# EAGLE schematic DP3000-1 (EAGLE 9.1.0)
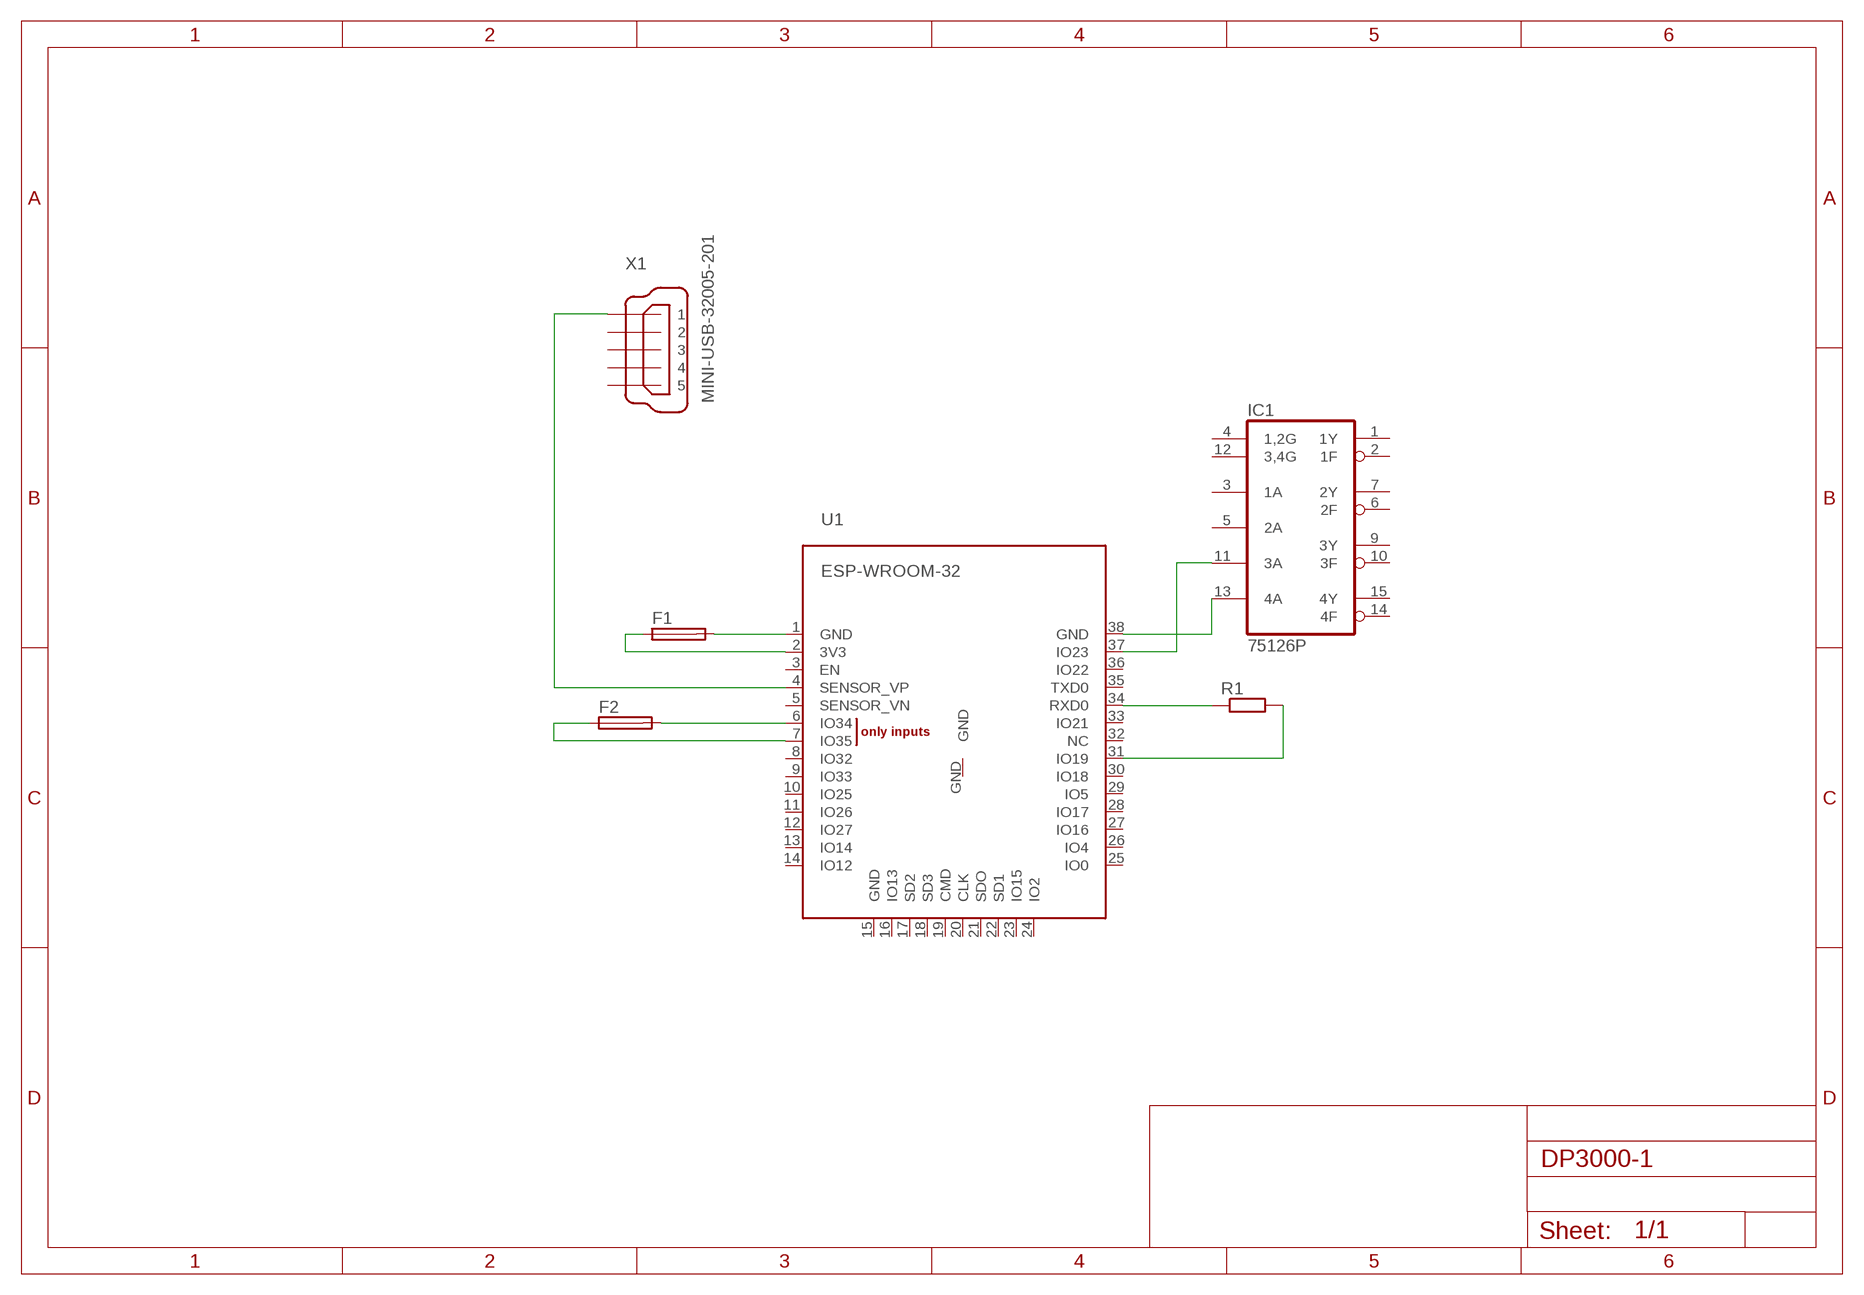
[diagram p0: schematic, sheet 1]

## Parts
F1  19560  [19560]
F2  KS16  [KS16]
IC1  75126P  [DIL16]
R1  R-EU_R2012  [R2012]
U1  ESP-WROOM-32  [ESP-WROOM-32]
X1  MINI-USB-32005-201  [32005-201]

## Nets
N$1: R1.1 U1.34(RXD0)
N$2: R1.2 U1.31(IO19)
N$3: IC1.13(4A) U1.38(GND)
N$4: IC1.11(3A) U1.37(IO23)
N$5: F1.2 U1.1(GND)
N$6: F1.1 U1.2(3V3)
N$7: F2.2 U1.6(IO34)
N$8: F2.1 U1.7(IO35)
N$9: U1.4(SENSOR_VP) X1.1
Unconnected: IC1.1(1Y) IC1.2(1F) IC1.3(1A) IC1.4(1,2G) IC1.5(2A) IC1.6(2F) IC1.7(2Y) IC1.9(3Y) IC1.10(3F) IC1.12(3,4G) IC1.14(4F) IC1.15(4Y) U1.3(EN) U1.5(SENSOR_VN) U1.8(IO32) U1.9(IO33) U1.10(IO25) U1.11(IO26) U1.12(IO27) U1.13(IO14) U1.14(IO12) U1.15(GND) U1.16(IO13) U1.17(SD2) U1.18(SD3) U1.19(CMD) U1.20(CLK) U1.21(SDO) U1.22(SD1) U1.23(IO15) U1.24(IO2) U1.25(IO0) U1.26(IO4) U1.27(IO16) U1.28(IO17) U1.29(IO5) U1.30(IO18) U1.32(NC) U1.33(IO21) U1.35(TXD0) U1.36(IO22) U1.GND X1.2 X1.3 X1.4 X1.5

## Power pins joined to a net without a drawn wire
GND: IC1.8(GND)
VCC: IC1.16(VCC)

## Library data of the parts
F1 = fuse:19560: FUSE HOLDER; MPN: 56000001009; OC_FARNELL: 1185363; OC_NEWARK: 15P8392
F2 = fuse:KS16: FUSE HOLDER; OC_FARNELL: unknown; OC_NEWARK: unknown
IC1 = 751xx:75126: 75xxx DEVICE
R1 = resistor:R-EU_: RESISTOR, European symbol
U1 = esp32:ESP-WROOM-32
X1 = con-cypressindustries:MINI-USB-: MINI USB-B Conector Source: www.cypressindustries.com; OC_FARNELL: unknown; OC_NEWARK: unknown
